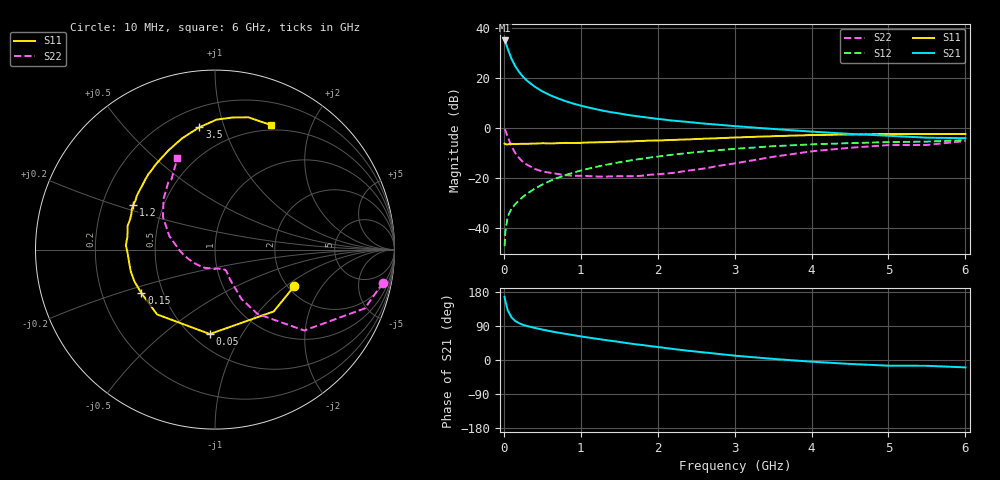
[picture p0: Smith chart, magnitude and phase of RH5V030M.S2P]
! SIEMENS Small Signal Semiconductors
! BFR106
! Si NPN RF Bipolar Junction Transistor in SOT23
! VCE = 5 V  IC = 30 mA
! Common Emitter S-Parameters:  August  1996
# GHz  S  MA  R  50
!  f  S11  S21  S12  S22
! GHz  MAG  ANG  MAG  ANG  MAG  ANG  MAG  ANG
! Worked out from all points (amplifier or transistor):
!   36 points, 10 MHz to 6 GHz, reference 50 ohm
!   highest |S21| = 35.1 dB at 10 MHz (marker M1)
!   |S21| within 3 dB of that: start of sweep to 46.65 MHz
!   unconditionally stable (mu >= 1): 312.5 MHz to 2.208 GHz
!   at 250 MHz: K = 0.95, MSG = 24.0 dB, |S12| = -27.5 dB
!   at 1.4 GHz: K = 1.06, MAG = 8.8 dB, |S12| = -14.3 dB
!   at 6 GHz: K = 0.99, MSG = 0.4 dB, |S12| = -4.9 dB
!   S11 on the Smith chart (normalised r, x): 10 MHz: 2.17, -1.15; 50 MHz: 0.61, -0.74; 150 MHz: 0.38, -0.24; 1.2 GHz: 0.33, +0.23; 3.5 GHz: 0.32, +0.83; 6 GHz: 0.44, +1.45
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0.01  0.487 -24.6  56.95 166.5  0.0043 82.2  0.9543 -11.1
0.02  0.4751 -46.5  53.01 155.6  0.0084 74.2  0.897 -21.4
0.05  0.4714 -93.5  38.95 131.4  0.0169 60.7  0.6711 -42.2
0.1  0.4843 -131.8  24.41 112.3  0.0244 57.4  0.4296 -56.5
0.15  0.4763 -149.5  17.15 102.6  0.0301 58.7  0.3127 -61.8
0.2  0.4829 -158.6  13.21 97.1  0.0359 61.9  0.2502 -62.3
0.25  0.4847 -165.7  10.63 92.7  0.042 63.8  0.2082 -62.9
0.3  0.4837 -170.5  8.934 89.8  0.0484 65.7  0.1855 -63.3
0.4  0.4872 -177.5  6.781 84.8  0.061 68.1  0.1523 -62.5
0.5  0.4972 177.2  5.443 80.3  0.0737 68.8  0.1355 -62.2
0.6  0.4933 172.3  4.569 76.2  0.0873 69.1  0.1272 -63.2
0.7  0.4974 168.1  3.946 72.4  0.1006 68.9  0.1204 -65.8
0.9  0.502 161.1  3.102 65.7  0.1275 67.6  0.1107 -69.4
1.1  0.5148 154.3  2.582 59.2  0.1538 65.8  0.1092 -78.0
1.2  0.5197 151.1  2.385 56.2  0.1672 64.7  0.1071 -81.9
1.6  0.5377 139.8  1.844 44.6  0.2191 59.7  0.1085 -101.7
2.2  0.5784 124.7  1.409 29.2  0.2939 51.6  0.1263 -136.2
3  0.6469 106.4  1.094 11.5  0.3833 39.7  0.196 -177.9
3.5  0.6872 97.3  0.959 2.9  0.4328 32.2  0.2653 163.5
4.5  0.7423 82.5  0.764 -10.4  0.4995 17.2  0.4025 135.5
5.5  0.7574 70.2  0.642 -15.3  0.5364 7.0  0.459 122.0
6  0.7613 65.9  0.627 -19.5  0.5709 -0.3  0.5499 112.4
